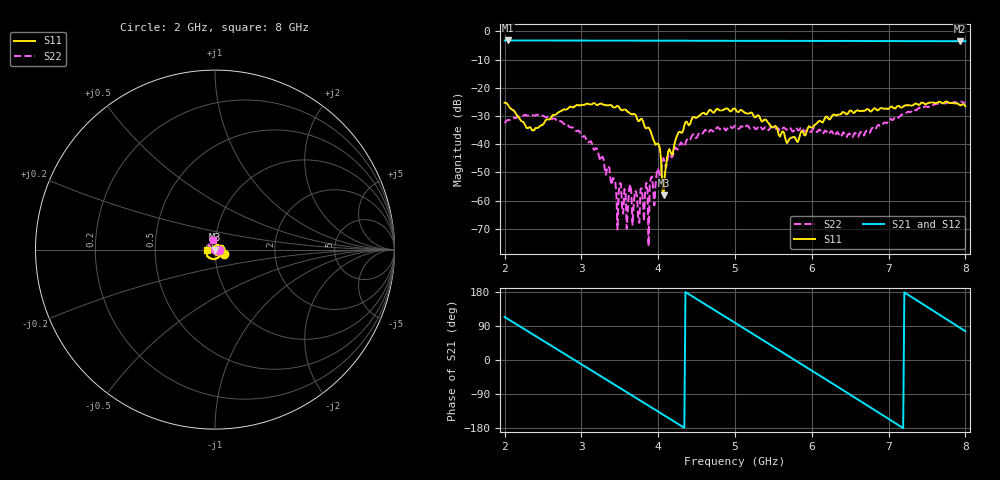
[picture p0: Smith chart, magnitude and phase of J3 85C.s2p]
!Agilent Technologies,E8364B,MY43040699,A.07.50.67
!Agilent E8364B: A.07.50.67
!Date: Friday, June 06, 2025 09:27:00
!Correction: S11(Full 2 Port(1,2))
!S21(Full 2 Port(1,2))
!S12(Full 2 Port(1,2))
!S22(Full 2 Port(1,2))
!S2P File: Measurements: S11, S21, S12, S22:
# Hz S  dB  R 50
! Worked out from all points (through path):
!   401 points, 2 GHz to 8 GHz, reference 50 ohm
!   highest |S21| = -3.19 dB at 2.045 GHz (marker M1); lowest = -3.5 dB at 7.925 GHz (marker M2)
!   group delay of S21, straight-line fit = 350 ps
!   lowest |S11| = -58.1 dB at 4.07 GHz (marker M3), VSWR 1.00, Z = 50 - j0.121 ohm
!   |S11| at or under -10 dB: start of sweep to end of sweep
!   |S22| runs from -76.2 to -24.9 dB; largest |S21 - S12| = 0.0065
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2e9  -25.30 -27.6  -3.20 113.5  -3.21 113.7  -32.48 -8.6
2.045e9  -26.05 -31.8  -3.19 107.9  -3.20 108.1  -31.39 -15.1
2.375e9  -35.16 9.6  -3.20 66.7  -3.22 66.7  -29.84 -48.9
2.705e9  -28.64 35.9  -3.23 25.5  -3.24 25.6  -31.80 -84.2
3.005e9  -26.04 15.9  -3.24 -11.9  -3.27 -11.9  -37.22 -118.0
3.26e9  -25.57 -6.9  -3.24 -43.7  -3.28 -43.6  -44.72 -139.4
3.56e9  -27.69 -35.5  -3.26 -81.1  -3.31 -81.0  -55.88 -49.0
3.815e9  -33.06 -71.8  -3.27 -113.1  -3.31 -112.9  -67.35 90.0
3.845e9  -34.41 -66.1  -3.26 -116.8  -3.31 -116.6  -53.67 53.7
4.01e9  -40.42 -105.9  -3.26 -137.5  -3.32 -137.3  -50.00 64.7
4.07e9  -58.13 -77.1  -3.27 -145.0  -3.32 -144.7  -44.92 88.4
4.13e9  -42.65 129.7  -3.28 -152.6  -3.33 -152.2  -44.08 91.4
4.355e9  -32.19 68.2  -3.29 179.2  -3.33 179.6  -39.74 61.4
5e9  -27.39 -24.3  -3.32 98.2  -3.34 98.7  -33.38 -28.9
5.315e9  -30.06 -72.5  -3.33 58.6  -3.34 59.0  -33.54 -81.7
5.69e9  -39.13 -165.0  -3.35 11.2  -3.35 11.7  -34.59 -140.1
6.005e9  -34.10 79.5  -3.36 -28.6  -3.35 -28.3  -35.12 174.0
6.5e9  -28.01 5.4  -3.37 -91.5  -3.38 -91.2  -36.62 145.0
7.01e9  -27.21 -47.1  -3.41 -156.7  -3.40 -156.5  -31.20 161.1
7.415e9  -25.64 -90.1  -3.43 151.4  -3.41 151.6  -27.10 139.2
7.925e9  -26.10 -162.9  -3.47 85.6  -3.43 85.8  -25.06 105.0
8e9  -26.53 -176.0  -3.46 76.0  -3.43 76.1  -25.15 99.9
